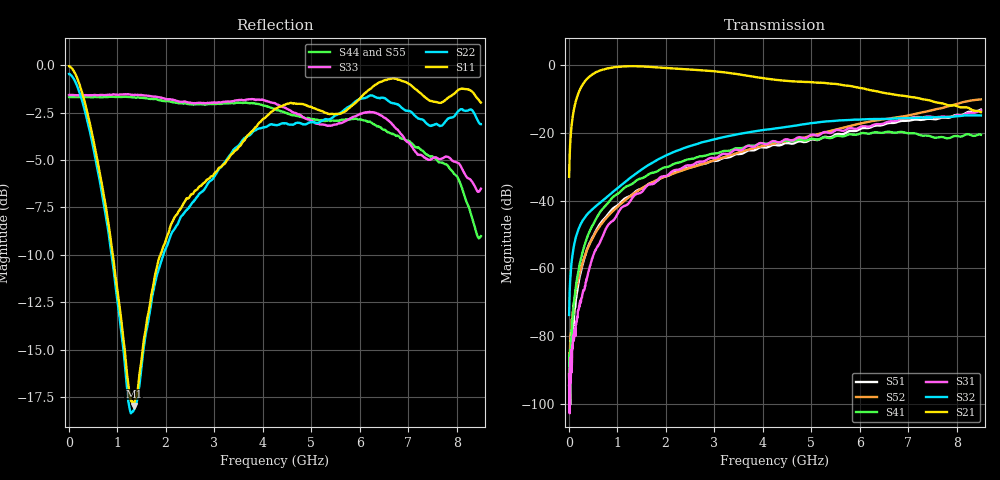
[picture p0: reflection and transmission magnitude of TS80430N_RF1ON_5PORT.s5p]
!Created with skrf (http://scikit-rf.org).
# GHz S RI R 50.0
!freq ReS11 ImS11 ReS12 ImS12 ReS13 ImS13
! ReS14 ImS14 ReS15 ImS15
! ReS21 ImS21 ReS22 ImS22 ReS23 ImS23
! ReS24 ImS24 ReS25 ImS25
! ReS31 ImS31 ReS32 ImS32 ReS33 ImS33
! ReS34 ImS34 ReS35 ImS35
! ReS41 ImS41 ReS42 ImS42 ReS43 ImS43
! ReS44 ImS44 ReS45 ImS45
! ReS51 ImS51 ReS52 ImS52 ReS53 ImS53
! ReS54 ImS54 ReS55 ImS55
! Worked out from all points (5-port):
!   1601 points, 10 MHz to 8.5 GHz, reference 50 ohm
!   strongest paths, dB at 10 MHz, 2.132 GHz, 4.255 GHz, 6.378 GHz, 8.5 GHz:
!     S21: -33.0, -1.0, -4.3, -7.8, -13.9
!     S32: -73.8, -25.9, -18.7, -15.9, -14.9
!     S31: -91.2, -31.4, -22.5, -17.4, -13.4
!     S41: -92.2, -29.4, -22.7, -19.9, -20.6
!     S52: -91.6, -32.2, -23.1, -16.3, -10.1
!     S51: -94.7, -32.1, -23.6, -17.8, -13.1
!   lowest |S11| = -18.0 dB at 1.342 GHz (marker M1), VSWR 1.29, Z = 39 + j2.55 ohm
!   |S11| at or under -10 dB: 912.8 MHz to 1.894 GHz (981.2 MHz wide, 69.9 % of centre)
